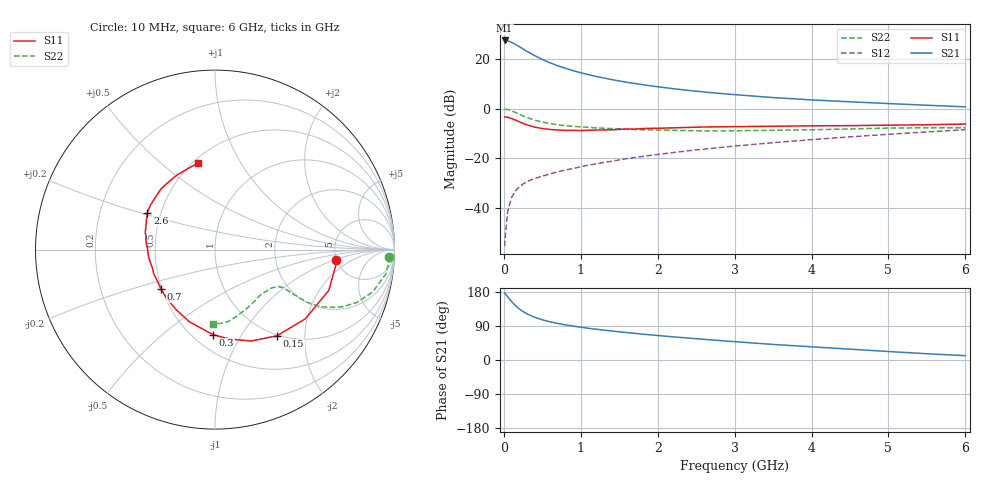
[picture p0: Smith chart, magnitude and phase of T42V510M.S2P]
! Infineon Technologies  Discrete & RF Semiconductors
! BFR182T
! Si NPN RF Bipolar Junction Transistor in SC75
! VCE = 2.5 V  IC = 10 mA
! Common Emitter S-Parameters:  October  1999
# GHz  S  MA  R  50
!  f  S11  S21  S12  S22
! GHz  MAG  ANG  MAG  ANG  MAG  ANG  MAG  ANG
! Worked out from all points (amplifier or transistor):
!   36 points, 10 MHz to 6 GHz, reference 50 ohm
!   highest |S21| = 27.5 dB at 10 MHz (marker M1)
!   |S21| within 3 dB of that: start of sweep to 227.3 MHz
!   unconditionally stable (mu >= 1): 957.8 MHz to 3.79 GHz
!   at 250 MHz: K = 0.46, MSG = 27.2 dB, |S12| = -30.3 dB
!   at 1.4 GHz: K = 1.09, MAG = 14.7 dB, |S12| = -21.2 dB
!   at 6 GHz: K = 0.84, MSG = 4.6 dB, |S12| = -8.4 dB
!   lowest NFmin = 1.50 dB at 450 MHz
!   S11 on the Smith chart (normalised r, x): 10 MHz: 4.95, -1.10; 150 MHz: 0.99, -1.46; 300 MHz: 0.62, -0.76; 700 MHz: 0.49, -0.25; 2.6 GHz: 0.42, +0.21; 6 GHz: 0.53, +0.68
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0.01  0.6775 -5.1  23.77 176.3  0.0017 81.2  0.9727 -2.4
0.02  0.6807 -6.6  23.59 174.8  0.0029 94.7  0.9741 -3.1
0.05  0.6734 -19.8  23.34 166.5  0.0085 85.6  0.9619 -8.0
0.1  0.634 -37.5  21.81 154.6  0.0162 74.7  0.9094 -15.1
0.15  0.5914 -54.3  19.88 143.7  0.022 68.1  0.8425 -20.5
0.2  0.5477 -68.4  17.89 135.0  0.0267 65.9  0.7781 -24.2
0.25  0.5059 -80.5  15.99 127.9  0.0304 60.7  0.7158 -26.7
0.3  0.474 -91.4  14.34 122.0  0.0341 59.5  0.6676 -28.4
0.4  0.4265 -109.6  11.77 112.7  0.0393 57.8  0.5886 -29.8
0.5  0.3982 -123.2  9.855 106.1  0.0438 58.1  0.5384 -29.7
0.6  0.3822 -134.7  8.424 100.8  0.0485 59.5  0.5028 -29.6
0.7  0.373 -143.6  7.371 96.5  0.0538 60.0  0.4755 -29.4
0.9  0.3669 -158.4  5.852 89.5  0.0624 62.0  0.4408 -29.2
1.1  0.3678 -169.5  4.864 83.6  0.0729 63.6  0.4207 -29.8
1.3  0.3744 -178.1  4.162 78.8  0.0828 64.5  0.4045 -30.8
1.6  0.389 171.8  3.413 72.3  0.0986 65.8  0.3876 -32.9
2.2  0.4125 158.4  2.537 61.1  0.1309 66.6  0.3674 -39.5
2.6  0.4288 151.4  2.178 54.5  0.1535 66.2  0.3592 -44.6
3.5  0.4428 137.8  1.679 41.1  0.2066 63.8  0.3677 -57.3
4.5  0.4566 124.8  1.379 28.6  0.271 59.3  0.3912 -72.5
5.5  0.4756 108.5  1.176 16.5  0.3416 53.7  0.4125 -85.6
6  0.492 100.8  1.092 11.4  0.3789 50.0  0.4121 -91.2
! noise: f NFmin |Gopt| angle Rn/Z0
0.45  1.5  0.26  43  0.28
0.9  1.6  0.24  87  0.22
1.8  2.1  0.2  170  0.2
